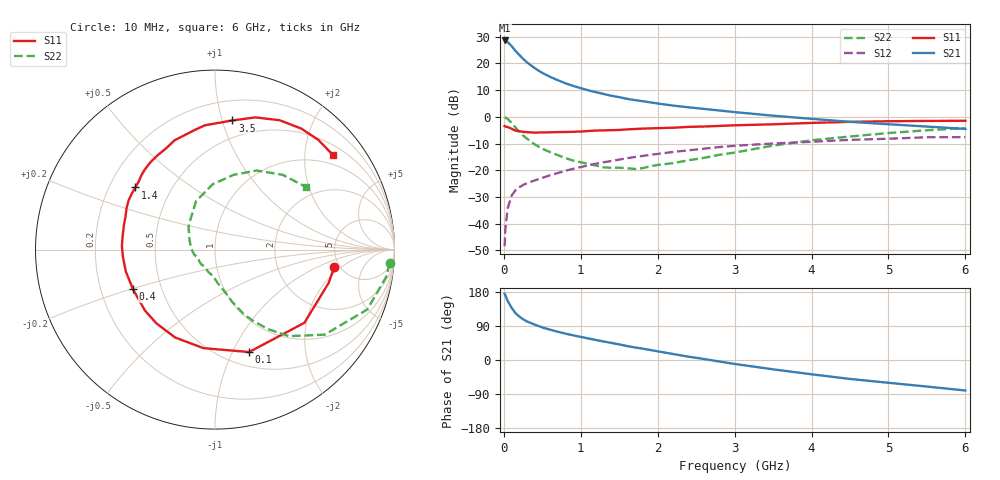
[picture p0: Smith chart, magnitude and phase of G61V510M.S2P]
! SIEMENS Small Signal Semiconductors
! BFG193
! Si NPN RF Bipolar Junction Transistor in SOT223
! VCE = 1.5 V  IC = 10 mA
! Common Emitter S-Parameters:  August  1996
# GHz  S  MA  R  50
!  f  S11  S21  S12  S22
! GHz  MAG  ANG  MAG  ANG  MAG  ANG  MAG  ANG
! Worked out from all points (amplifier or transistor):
!   36 points, 10 MHz to 6 GHz, reference 50 ohm
!   highest |S21| = 28.6 dB at 10 MHz (marker M1)
!   |S21| within 3 dB of that: start of sweep to 126.2 MHz
!   unconditionally stable (mu >= 1): 847.2 MHz to 2.774 GHz
!   at 250 MHz: K = 0.54, MSG = 23.6 dB, |S12| = -25.5 dB
!   at 1.4 GHz: K = 1.08, MAG = 10.5 dB, |S12| = -16.5 dB
!   at 6 GHz: K = 0.93, MSG = 1.5 dB, |S12| = -7.6 dB
!   S11 on the Smith chart (normalised r, x): 10 MHz: 4.52, -1.58; 100 MHz: 0.65, -1.16; 400 MHz: 0.34, -0.20; 1.4 GHz: 0.31, +0.31; 3.5 GHz: 0.35, +1.08; 6 GHz: 0.74, +2.68
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0.01  0.6717 -8.2  26.91 174.8  0.0038 88.2  0.9765 -4.5
0.02  0.6602 -16.3  26.66 170.6  0.0081 83.3  0.9663 -9.0
0.05  0.6437 -39.3  25.05 155.6  0.0194 73.4  0.9114 -21.5
0.1  0.6016 -71.6  21.19 138.3  0.0333 60.8  0.7734 -37.8
0.15  0.5526 -96.8  17.29 123.9  0.0422 53.0  0.6339 -49.5
0.2  0.5378 -114.4  14.46 114.9  0.0481 50.0  0.532 -56.3
0.25  0.5249 -128.4  12.19 107.5  0.0531 47.7  0.4486 -62.0
0.3  0.5173 -139.0  10.52 101.8  0.0573 47.1  0.392 -66.1
0.4  0.5076 -154.2  8.184 93.4  0.0645 46.8  0.3064 -71.8
0.5  0.5117 -166.2  6.638 85.9  0.0723 46.8  0.2527 -75.8
0.6  0.5142 -174.9  5.621 80.1  0.0808 47.8  0.219 -79.8
0.7  0.5191 177.8  4.861 74.6  0.0888 47.8  0.1925 -84.4
0.9  0.5255 164.9  3.807 65.1  0.1065 47.1  0.152 -92.6
1.1  0.543 155.3  3.135 56.8  0.1237 45.8  0.1324 -105.1
1.4  0.5634 142.1  2.478 45.0  0.1492 42.1  0.1112 -126.8
1.7  0.5921 131.6  2.063 33.2  0.1768 37.7  0.1058 -151.5
2.2  0.6265 115.8  1.625 15.9  0.2202 28.1  0.1361 172.9
2.8  0.6768 99.4  1.316 -4.0  0.2718 15.5  0.1945 139.3
3.5  0.7262 82.3  1.052 -24.6  0.3173 -0.9  0.2905 111.2
4.5  0.8056 63.5  0.808 -50.0  0.3713 -20.4  0.4294 76.0
5.5  0.8395 46.8  0.658 -70.1  0.4149 -43.5  0.5618 47.9
6  0.843 38.5  0.595 -80.5  0.4175 -56.8  0.6154 34.5
